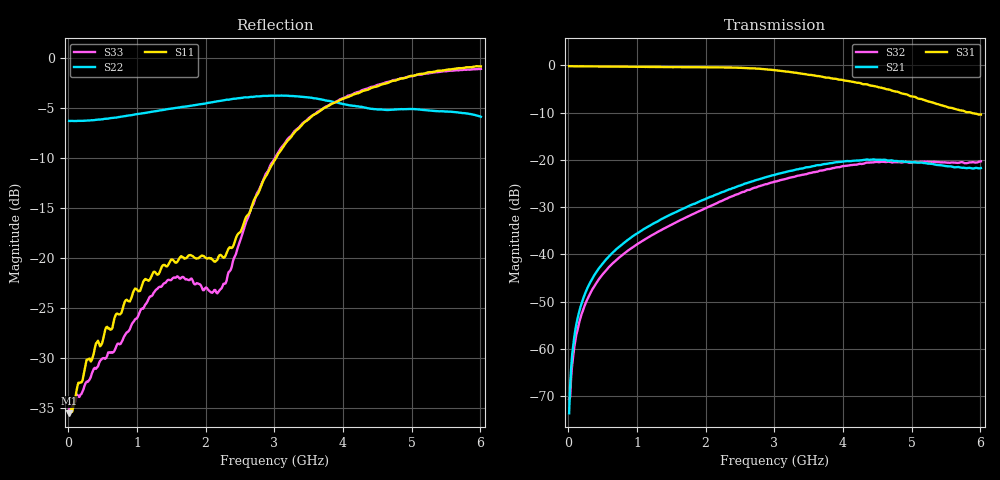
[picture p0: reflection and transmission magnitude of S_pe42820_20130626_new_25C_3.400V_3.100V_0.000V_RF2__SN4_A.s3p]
! Device ID: pe42820_20130626_new
! Dir: c:\SVN\PSC 4Port_VNA Bench\CVI 2009\branches\PE42820\pe42820_matching\pe42820_20130626_new\25C\3p400000\RF2
! Serial: 4
! Insertion: A
! Temp: 25C
! VDD: 3.400
! Control_Hi: 3.100
! Control_Lo: 0.000
! Logic State: RF2
! ThroughPath: 3-1
! Port 1: RFC
! Port 2: RF1
! Port 3: RF2
! V1 = 0.00
! V2 = 0.00
! V3 = 0.00
! IDD: 1.341070e-04
! FILE NAME
! DATE 06/27/13  15:32
! CORRECTED  DATA
#  Hz  S  RI  R  50
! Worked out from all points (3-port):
!   401 points, 10 MHz to 6.01 GHz, reference 50 ohm
!   strongest paths, dB at 10 MHz, 1.51 GHz, 3.01 GHz, 4.51 GHz, 6.01 GHz:
!     S31: -0.2, -0.4, -1.0, -4.6, -10.4
!     S21: -73.6, -31.4, -23.1, -20.0, -21.7
!     S32: -70.7, -33.7, -24.6, -20.4, -20.3
!   lowest |S11| = -35.5 dB at 10 MHz (marker M1), VSWR 1.03, Z = 51.7 + j0.19 ohm
!   |S11| at or under -10 dB: start of sweep to 3.023 GHz
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1e7  0.0166 0.00184  5.95e-05 7.85e-05  0.9803 -0.00602
     8.96e-05 0.000188  -0.4868 0.00626  0.000222 0.000183
     0.9823 -0.00754  0.000165 0.000243  0.0174 0.00219
7e7  0.0175 0.00439  0.00013 0.00108  0.9778 -0.0561
     0.000143 0.00109  -0.4847 0.0397  0.000108 0.000848
     0.9794 -0.0575  0.00014 0.000842  0.0178 0.00526
1.45e8  0.0221 0.00872  0.000249 0.00227  0.972 -0.1142
        0.000239 0.00228  -0.4803 0.079  0.000224 0.00175
        0.9708 -0.1148  0.000218 0.00174  0.0181 0.0091
5.2e8  0.0404 0.00905  0.0023 0.00808  0.8912 -0.3936
       0.00227 0.00805  -0.4207 0.2667  0.00165 0.00621
       0.8909 -0.3949  0.00166 0.0062  0.0208 0.0238
1.885e9  0.0281 -0.0958  0.0305 0.0178  0.0573 -0.9535
         0.0307 0.0182  0.0986 0.5786  0.0228 0.0169
         0.0583 -0.9554  0.0227 0.0168  0.0321 0.0675
2.275e9  -0.0638 -0.0781  0.0448 0.0128  -0.256 -0.9184
         0.0448 0.0124  0.2435 0.5681  0.0352 0.0144
         -0.2587 -0.9151  0.0352 0.0146  -0.0158 0.0728
3.01e9  -0.2001 0.2377  0.0664 -0.0226  -0.7273 -0.5122
        0.0659 -0.0226  0.4422 0.4782  0.0575 -0.0118
        -0.7278 -0.5119  0.0577 -0.0119  -0.1473 0.2822
4.06e9  0.3397 0.5417  0.0265 -0.0938  -0.6557 0.2117
        0.0265 -0.0938  0.5405 0.2258  0.0396 -0.0775
        -0.655 0.2096  0.0398 -0.0773  0.139 0.6317
4.975e9  0.8129 0.0593  -0.051 -0.0795  -0.2371 0.4114
         -0.0519 -0.0794  0.557 0.0356  -0.0292 -0.0894
         -0.2359 0.4132  -0.0288 -0.0888  0.5678 0.5823
6.01e9  0.7948 -0.4465  -0.0763 -0.0291  -0.00245 0.3014
        -0.0764 -0.0299  0.5074 -0.0546  -0.0778 -0.0572
        -0.00282 0.3027  -0.0782 -0.0569  0.8387 0.2864
